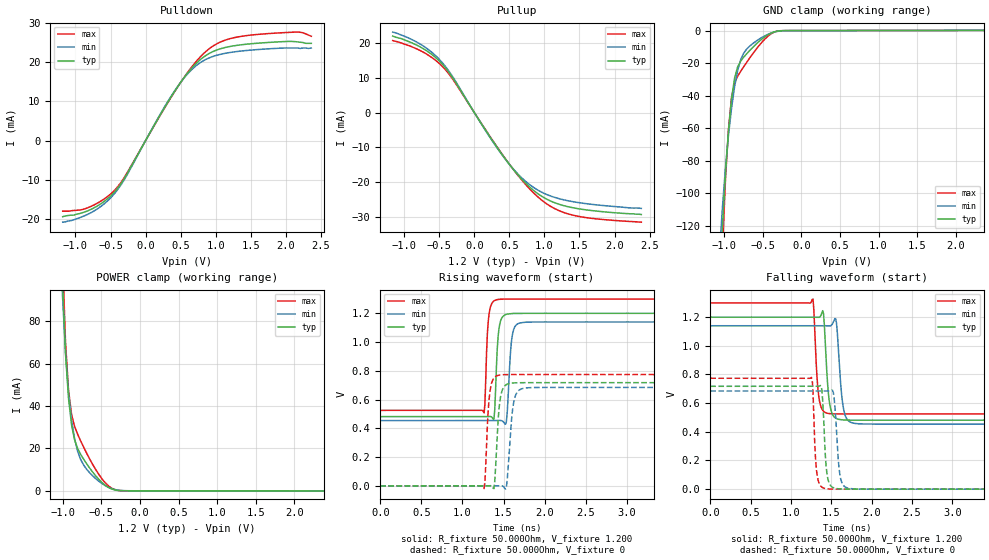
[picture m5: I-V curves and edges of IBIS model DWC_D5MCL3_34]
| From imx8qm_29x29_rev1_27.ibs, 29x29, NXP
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[Model] DWC_D5MCL3_34
Model_type   I/O
Polarity   Non-Inverting
Enable   Active-High
C_comp   1.264pF   1.181pF   1.367pF
C_comp_pullup   284.432fF   261.981fF   311.492fF
C_comp_pulldown 969.059fF   903.013fF   1.049pF
Vinh = 952.000mV
Vinl = 682.000mV
Vmeas = 817.000mV
Vref = 817.000mV
Rref = 50Ohms
Cref = 5pF
[Model Spec]
Vinh   952.000mV   911.000mV   1.020V
Vinl   682.000mV   641.000mV   750.000mV
Vmeas   817.000mV   776.000mV   885.000mV
Vref   817.000mV   776.000mV   885.000mV
D_overshoot_ampl_h 0.35 NA   NA
D_overshoot_ampl_l 0.35 NA   NA
D_overshoot_area_l 100.000p NA   NA
D_overshoot_area_h 100.000p NA   NA
[Receiver Thresholds]
Vth = 817.000mV
Vth_min = 805.000mV
Vth_max = 829.000mV
Vinh_ac = 135.000mV
Vinh_dc = 100.000mV
Vinl_ac = -135.000mV
Vinl_dc = -100.000mV
Tslew_ac = 5.000ns
Reference_supply Pullup_ref
[Temperature Range]   25.000   125.000   -40.000
[Voltage Range]   1.200V   1.140V   1.300V
[GND Clamp Reference]   0.00V   0.00V   0.00V
[C Comp Corner]
| variable   typ   min   max
C_comp 1.264pF   1.367pF   1.181pF
C_comp_pullup 284.432fF   311.492fF   261.981fF
C_comp_pulldown 969.059fF   1.049pF   903.013fF
[Pulldown Reference]   0.00V   0.00V   0.00V
[POWER Clamp Reference]   1.200V   1.140V   1.300V
[Pullup Reference]   1.200V   1.140V   1.300V
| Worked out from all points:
|   slope of the pulldown table from 0 to 0.18 V, typ, clamps not added: 31.8 ohm
|   slope of the pullup table from 0 to 0.18 V, typ, clamps not added: 31.9 ohm
|   GND clamp passes 1 mA (typ) near -0.36 V on its own axis
|   POWER clamp passes 1 mA (typ) near -0.38 V on its own axis
|   rising waveform, R_fixture 50.000Ohm, V_fixture 1.200: 20-80 % time 37.1ps typ, 43.2ps min, 34.3ps max; typ from 0.481 V to 1.2 V
|   rising waveform, R_fixture 50.000Ohm, V_fixture 0: 20-80 % time 47.7ps typ, 56.6ps min, 43.2ps max; typ from 0 V to 0.717 V
|   falling waveform, R_fixture 50.000Ohm, V_fixture 1.200: 20-80 % time 50.4ps typ, 57.7ps min, 46ps max; typ from 1.2 V to 0.481 V
|   falling waveform, R_fixture 50.000Ohm, V_fixture 0: 20-80 % time 41.7ps typ, 49.9ps min, 36ps max; typ from 0.717 V to 0 V
[GND Clamp]
-1.182V   -339.3mA   -254.8mA   -426.6mA
-1.064V   -163.5mA   -137.8mA   -190.4mA
-1.024V   -121.1mA   -108.6mA   -134.3mA
-984.8mV  -87.5mA    -84.22mA   -91.46mA
-945.5mV  -61.36mA   -64.12mA   -60.5mA
-906.1mV  -41.91mA   -47.62mA   -41.1mA
-866.7mV  -29.17mA   -34.43mA   -32.17mA
-827.3mV  -22.35mA   -24.56mA   -28.07mA
-748.5mV  -16.34mA   -13.87mA   -22.22mA
-590.9mV  -8.454mA   -6.602mA   -11.71mA
-275.8mV  -116.4uA   -248.8uA   -84.78uA
2.364V    136.6uA    111.3uA    170.2uA
[Power Clamp]
-1.164V   362.5mA    268.1mA    465.2mA
-1.006V   98.99mA    92.43mA    111.8mA
-966.7mV  64.74mA    65.63mA    70.25mA
-927.3mV  43.55mA    46.45mA    47.41mA
-887.9mV  31.08mA    33.31mA    36.05mA
-848.5mV  24.04mA    24.48mA    30.35mA
-809.1mV  19.97mA    18.62mA    26.67mA
-690.9mV  12.66mA    10.09mA    17.63mA
-493.9mV  3.911mA    3.404mA    5.643mA
-375.8mV  976.4uA    1.116mA    1.399mA
-257.6mV  56.8uA     160.4uA    65.6uA
2.382V    -68.29uA   -58.74uA   -77.9uA
[Pulldown]
-1.182V   -19.4mA    -20.8mA    -18mA
-827.3mV  -17.92mA   -18.81mA   -17.15mA
-630.3mV  -16.01mA   -16.68mA   -15.35mA
-433.3mV  -12.9mA    -13.29mA   -12.49mA
-275.8mV  -8.812mA   -9.115mA   -8.565mA
354.5mV   10.88mA    11.04mA    10.75mA
551.5mV   16.11mA    16.02mA    16.17mA
748.5mV   20.13mA    19.47mA    20.72mA
984.8mV   22.88mA    21.59mA    24.36mA
1.3V      24.27mA    22.7mA     26.37mA
2.167V    25.17mA    23.6mA     27.66mA
2.364V    24.8mA     23.6mA     26.6mA
[Pullup]
-1.164V   21.9mA     23.05mA    20.61mA
-730.3mV  18.32mA    19.1mA     17.32mA
-572.7mV  16.1mA     16.67mA    15.27mA
-415.1mV  12.89mA    13.27mA    12.34mA
-297mV    9.589mA    9.909mA    9.243mA
372.7mV   -11.36mA   -11.48mA   -11.23mA
609.1mV   -17.54mA   -17.33mA   -17.66mA
806.1mV   -21.63mA   -20.9mA    -22.22mA
1.042V    -24.91mA   -23.55mA   -26.28mA
1.318V    -26.88mA   -25.18mA   -28.9mA
1.673V    -28.06mA   -26.28mA   -30.3mA
2.382V    -29.2mA    -27.45mA   -31.4mA
[Ramp]
R_load=50.000Ohm
dV/dt_r   430.380mV/43.000ps  410.819mV/51.000ps  464.040mV/39.000ps
dV/dt_f   430.380mV/46.500ps  410.819mV/54.500ps  464.040mV/41.500ps
[Rising waveform]
R_fixture=50.000Ohm
V_fixture=1.200
V_fixture_min=1.140
V_fixture_max=1.300
0s        481.2mV    453.7mV    524.6mV
1.263ns   481.2mV    453.7mV    507mV
1.303ns   481.2mV    453.7mV    1.054V
1.323ns   482mV      453.7mV    1.191V
1.383ns   463.6mV    453.6mV    1.285V
1.444ns   1.09V      455mV      1.296V
1.534ns   1.192V     445.5mV    1.298V
1.614ns   1.198V     1.067V     1.298V
1.744ns   1.199V     1.136V     1.298V
10ns      1.199V     1.139V     1.298V
[Rising waveform]
R_fixture=50.000Ohm
V_fixture=0
0s        168.4nV    4.199uV    23.43nV
1.263ns   -5.66uV    3.088uV    -18.82mV
1.333ns   1.287mV    14.46uV    648mV
1.383ns   -19.04mV   -102.6uV   749mV
1.464ns   619mV      1.651mV    771.1mV
1.534ns   703.6mV    -9.729mV   773.2mV
1.594ns   713.8mV    438.9mV    773.5mV
1.634ns   715.8mV    606.8mV    773.5mV
1.764ns   717.2mV    679.8mV    773.6mV
10ns      717.1mV    684.1mV    773.2mV
[Falling waveform]
R_fixture=50.000Ohm
V_fixture=1.200
V_fixture_min=1.140
V_fixture_max=1.300
0s        1.199V     1.139V     1.298V
1.273ns   1.199V     1.139V     1.325V
1.333ns   1.198V     1.139V     702.3mV
1.403ns   1.224V     1.139V     543.1mV
1.474ns   614.8mV    1.138V     526.7mV
1.554ns   494.9mV    1.188V     524.4mV
1.624ns   483.8mV    677.7mV    524.2mV
1.654ns   482.4mV    551.5mV    524.1mV
1.794ns   481mV      458mV      524.1mV
10ns      481.1mV    453.7mV    524.5mV
[Falling waveform]
R_fixture=50.000Ohm
V_fixture=0
0s        717mV      684.1mV    773.1mV
1.253ns   717mV      684.1mV    778.9mV
1.273ns   717mV      684.1mV    672.3mV
1.323ns   716.6mV    684.1mV    101mV
1.383ns   689.5mV    684.1mV    13.74mV
1.444ns   114.9mV    683.6mV    2.499mV
1.524ns   10.23mV    675.3mV    302.3uV
1.614ns   1.415mV    76.66mV    31.83uV
1.734ns   121.2uV    4.332mV    7.596uV
10ns      505.9nV    4.365uV    318.7nV
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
